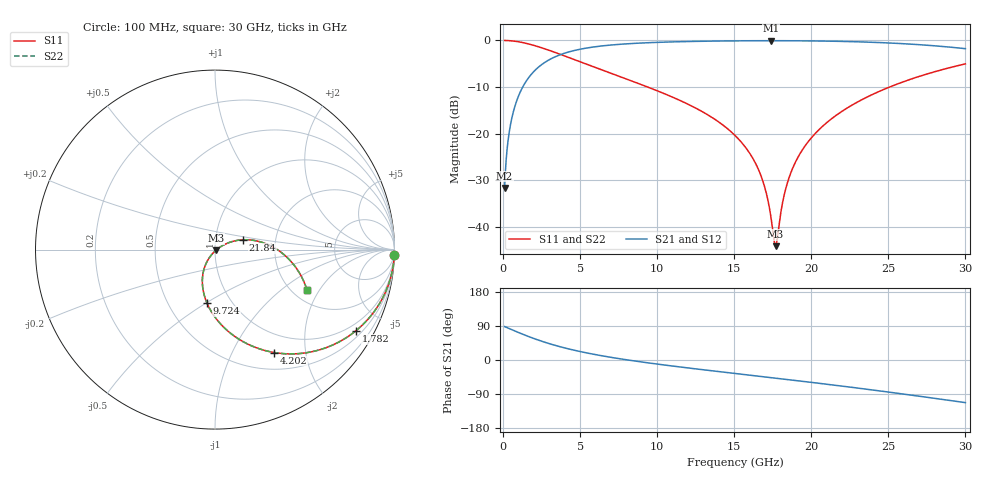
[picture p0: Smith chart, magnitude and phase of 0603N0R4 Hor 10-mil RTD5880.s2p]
# GHz S MA R 50
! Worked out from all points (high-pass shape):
!   3201 points, 100 MHz to 30 GHz, reference 50 ohm
!   highest |S21| = -0.06 dB at 17.4 GHz (marker M1); lowest = -31.7 dB at 100 MHz (marker M2)
!   |S21| within 3 dB of the highest: 3.714 GHz to end of sweep
!   lowest |S11| = -44.2 dB at 17.68 GHz (marker M3), VSWR 1.01, Z = 50.4 - j0.458 ohm
!   |S11| at or under -10 dB: 9.385 GHz to 25.08 GHz (15.7 GHz wide, 91.1 % of centre)
!   |S22| runs from -44.2 to 0.0 dB; largest |S21 - S12| = 0
!   S11 on the Smith chart (normalised r, x): 100 MHz: 1, -65; 1.782 GHz: 0.71, -3.60; 4.202 GHz: 0.72, -1.48; 9.724 GHz: 0.77, -0.50; 21.84 GHz: 1.36, +0.15; 30 GHz: 2.38, -1.56
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0.1  0.9997 -1.8  0.02607 88.2  0.02607 88.2  0.9997 -1.8
0.3709688  0.9953 -6.6  0.09632 83.4  0.09632 83.4  0.9953 -6.6
0.660625  0.9854 -11.6  0.1699 78.4  0.1699 78.4  0.9854 -11.6
1.127813  0.9591 -19.6  0.2827 70.4  0.2827 70.4  0.9591 -19.6
1.781875  0.9058 -30.0  0.4231 60.0  0.4231 60.0  0.9058 -30.0
2.86575  0.7964 -45.1  0.6035 44.8  0.6035 44.8  0.7964 -45.1
4.201906  0.6618 -60.1  0.7479 29.8  0.7479 29.8  0.6618 -60.1
5.089563  0.5828 -68.3  0.8105 21.5  0.8105 21.5  0.5828 -68.3
7.163875  0.4342 -83.7  0.8979 5.9  0.8979 5.9  0.4342 -83.7
9.724063  0.3007 -98.6  0.95 -9.3  0.95 -9.3  0.3007 -98.6
10.06978  0.2854 -100.4  0.9546 -11.1  0.9546 -11.1  0.2854 -100.4
15.05  0.0956 -122.4  0.99 -35.5  0.99 -35.5  0.0956 -122.4
16.58237  0.04082 -124.6  0.9932 -42.7  0.9932 -42.7  0.04082 -124.6
17.04956  0.02412 -120.6  0.9935 -44.9  0.9935 -44.9  0.02412 -120.6
17.39528  0.01227 -106.8  0.9936 -46.5  0.9936 -46.5  0.01227 -106.8
17.68494  0.006197 -47.1  0.9936 -47.9  0.9936 -47.9  0.006197 -47.1
18.20819  0.02074 21.7  0.9932 -50.4  0.9932 -50.4  0.02074 21.7
18.58194  0.03458 26.9  0.9926 -52.2  0.9926 -52.2  0.03458 26.9
20.03956  0.09154 26.4  0.9884 -59.2  0.9884 -59.2  0.09154 26.4
21.84291  0.167 19.2  0.9778 -68.1  0.9778 -68.1  0.167 19.2
25.01978  0.3133 3.6  0.9399 -84.7  0.9399 -84.7  0.3133 3.6
30  0.5602 -23.7  0.8161 -112.5  0.8161 -112.5  0.5602 -23.7
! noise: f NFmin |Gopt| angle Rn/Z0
0.1  0.0006395  0.9753  1.345  0.005892
3.417  0.003969  0.8094  10.92  0.004299
6.743  0.006666  0.7788  19.59  0.005995
10.06  0.009191  0.7637  28.32  0.007433
13.39  0.01175  0.7569  36.97  0.00881
16.7  0.01445  0.756  45.42  0.01022
20.03  0.01744  0.7599  53.71  0.01177
23.35  0.02084  0.7678  61.78  0.01354
26.67  0.02484  0.7793  69.67  0.01565
30  0.0297  0.7938  77.37  0.01828
